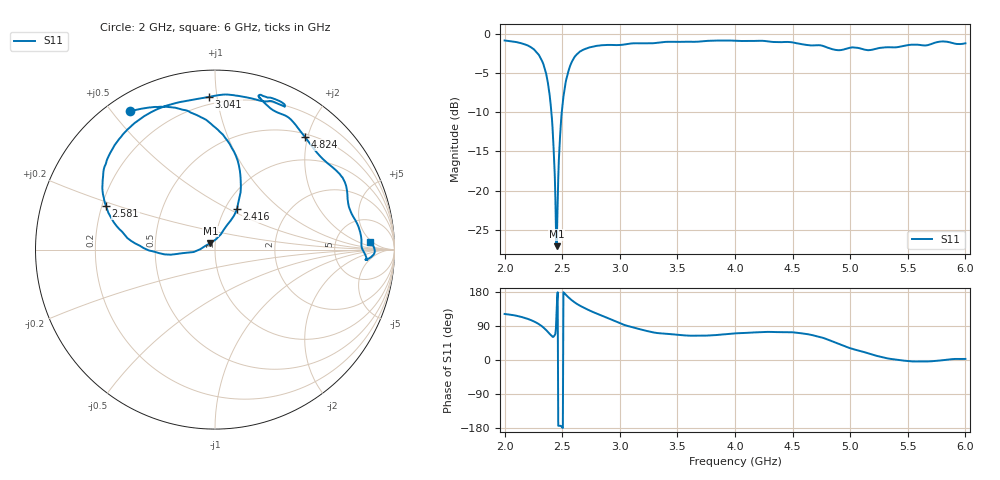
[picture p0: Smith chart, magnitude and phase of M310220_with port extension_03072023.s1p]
# Hz S RI R 50
! CMT, M5090, 19127454, 21.2.4/2
! Date: 3/7/2023 4:33:19 PM
! Data: Format (Calibration Info)
! Freq	S11:Re/Im(F2 Pxt)
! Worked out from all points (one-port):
!   800 points, 2 GHz to 6 GHz, reference 50 ohm
!   lowest |S11| = -27.0 dB at 2.451 GHz (marker M1), VSWR 1.09, Z = 47.4 + j3.48 ohm
!   |S11| at or under -10 dB: 2.406 GHz to 2.496 GHz (90.39 MHz wide, 3.69 % of centre)
!   S11 on the Smith chart (normalised r, x): 2 GHz: 0.07, +0.56; 2.416 GHz: 1.14, +0.55; 2.581 GHz: 0.22, +0.18; 3.041 GHz: 0.15, +0.95; 4.824 GHz: 0.55, +1.95; 6 GHz: 12, +4
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2e9  -0.4719 0.7701
2.155194e9  -0.3345 0.7948
2.285357e9  -0.0902 0.7441
2.365457e9  0.1173 0.5204
2.395494e9  0.1443 0.352
2.415519e9  0.1225 0.2248
2.435544e9  0.0512 0.1139
2.450563e9  -0.0251 0.0367
2.465582e9  -0.1189 -0.0135
2.485607e9  -0.2465 -0.0283
2.500626e9  -0.3385 -0.0115
2.530663e9  -0.4881 0.0641
2.580726e9  -0.6065 0.241
2.65582e9  -0.615 0.4631
2.760951e9  -0.5014 0.6548
3.001252e9  -0.1016 0.8392
3.041302e9  -0.0342 0.8507
3.296621e9  0.261 0.828
3.501877e9  0.3542 0.8112
3.747184e9  0.3886 0.8077
4.002503e9  0.3028 0.847
4.503129e9  0.2558 0.8392
4.733417e9  0.4081 0.7371
4.823529e9  0.5 0.6289
5.003755e9  0.6993 0.4153
5.30413e9  0.8128 0.0783
5.50438e9  0.8437 -0.0452
6e9  0.8651 0.043
